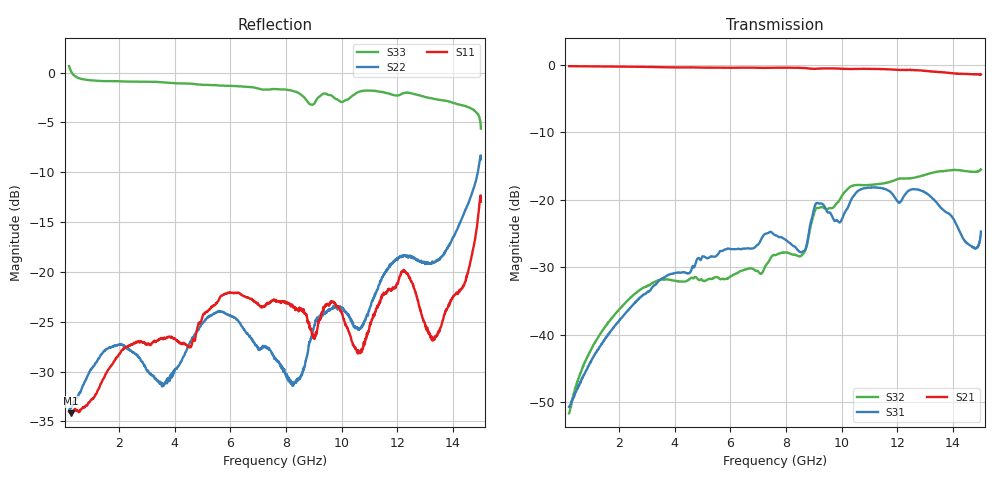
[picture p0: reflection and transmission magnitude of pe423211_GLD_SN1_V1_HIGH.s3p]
! Created Mon Jan 20 11:13:26 2025
# mhz S ri R 50
! 3 Port Network Data from SP1.SP block
! freq  reS11  imS11  reS12  imS12  reS13  imS13
!  reS21  imS21
!  reS22  imS22  reS23  imS23
!  reS31  imS31  reS32  imS32
!  reS33  imS33
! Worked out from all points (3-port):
!   1481 points, 200 MHz to 15 GHz, reference 50 ohm
!   strongest paths, dB at 200 MHz, 3.9 GHz, 7.6 GHz, 11.3 GHz, 15 GHz:
!     S21: -0.2, -0.4, -0.4, -0.6, -1.4
!     S31: -50.7, -31.0, -25.2, -18.2, -24.7
!     S32: -51.7, -32.0, -28.2, -17.7, -15.5
!   lowest |S11| = -34.2 dB at 260 MHz (marker M1), VSWR 1.04, Z = 52 + j0.0942 ohm
!   |S11| at or under -10 dB: start of sweep to end of sweep
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200  0.0199 6.12e-05  0.9759 -0.0326  0.00283 -0.000374
     0.976 -0.0324  0.0202 -0.000203  0.00177 0.00184
     0.00289 -0.000381  0.00177 0.00192  -0.419 -0.991
260  0.0195 0.000905  0.9753 -0.0432  0.0029 -0.000928
     0.9755 -0.0433  0.0207 0.000704  0.00181 0.00232
     0.00293 -0.000941  0.00185 0.0023  -0.6098 -0.8189
810  0.0183 0.0109  0.9642 -0.1356  0.0019 -0.00509
     0.9642 -0.1356  0.0276 0.00864  0.00272 0.00594
     0.00184 -0.00509  0.00267 0.00592  -0.9058 -0.1553
2160  0.0298 0.0288  0.9033 -0.3508  -0.00668 -0.0122
      0.9036 -0.3511  0.0345 0.025  0.00654 0.0153
      -0.00669 -0.0122  0.00655 0.0153  -0.8498 0.3022
7600  0.0393 -0.0608  0.2641 -0.9142  -0.0285 0.0467
      0.2635 -0.9141  -0.00318 0.0367  0.0171 0.0348
      -0.0285 0.0467  0.0172 0.0349  0.0223 0.8246
8600  0.0283 -0.0565  0.0922 -0.9429  -0.0259 0.0322
      0.0923 -0.9426  0.0193 0.0252  0.00727 0.039
      -0.0259 0.0323  0.00727 0.039  0.2002 0.7345
10620  -0.015 -0.0366  -0.2387 -0.9005  -0.00967 0.1172
       -0.2388 -0.9008  0.0298 0.0417  0.0983 0.0831
       -0.0098 0.1171  0.0981 0.0831  0.3444 0.7229
12240  -0.1015 -0.0024  -0.4903 -0.773  0.0569 0.0902
       -0.4905 -0.7737  -0.0425 0.1123  0.1404 0.0303
       0.0569 0.0902  0.1404 0.0303  0.5928 0.5191
13300  -0.000501 0.0457  -0.6198 -0.6372  0.0929 0.0382
       -0.6202 -0.6376  -0.0371 0.105  0.1586 -0.0124
       0.093 0.0383  0.1586 -0.0124  0.6372 0.3723
15000  -0.1113 0.1954  -0.7171 -0.4556  0.0152 0.0566
       -0.7157 -0.4552  -0.0991 0.3536  0.1106 -0.1254
       0.015 0.0561  0.1109 -0.1255  0.5024 0.1458
